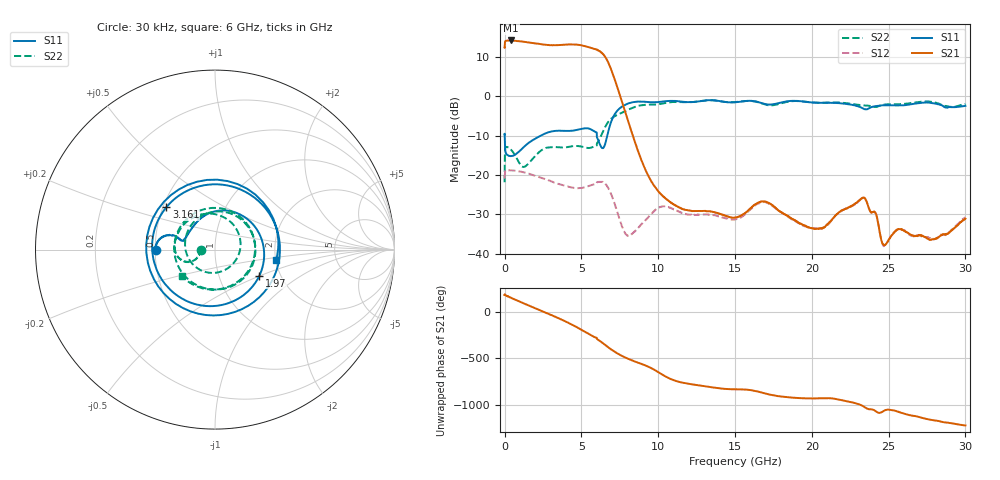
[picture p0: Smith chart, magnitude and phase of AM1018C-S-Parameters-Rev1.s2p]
# Hz S DB R 50.0
!freq dBS11 angS11 dBS21 angS21 dBS12 angS12 dBS22 angS22
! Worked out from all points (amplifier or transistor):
!   2882 points, 30 kHz to 30 GHz, reference 50 ohm
!   highest |S21| = 14.2 dB at 431.6 MHz (marker M1)
!   |S21| within 3 dB of that: start of sweep to 6.277 GHz
!   unconditionally stable (mu >= 1): start of sweep to end of sweep
!   at 1.168 MHz: K = 1.38, MAG = 12.8 dB, |S12| = -20.7 dB
!   at 1.784 GHz: K = 1.20, MAG = 14.0 dB, |S12| = -20.0 dB
!   at 30 GHz: K = 100.35, MAG = -23.2 dB, |S12| = -30.8 dB
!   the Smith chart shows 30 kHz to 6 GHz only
!   S11 on the Smith chart (normalised r, x): 30 kHz: 0.50, -0.00; 1.97 GHz: 1.56, -0.49; 3.161 GHz: 0.52, +0.28; 6 GHz: 2.00, -0.27
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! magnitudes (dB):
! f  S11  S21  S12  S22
! 30 kHz  -9.7  12.3  -20.7  -21.9
! 15.16 MHz  -11.6  13.4  -19.6  -15.0
! 40.55 MHz  -13.8  14.0  -19.0  -13.2
! 431.6 MHz  -15.2  14.2  -18.8  -13.6
! 1.191 GHz  -13.1  13.9  -19.3  -18.0
! 1.97 GHz  -10.8  13.4  -20.2  -15.3
! 3.161 GHz  -8.9  13.0  -21.8  -12.9
! 5.034 GHz  -8.3  12.9  -23.3  -12.8
! 6 GHz  -9.3  11.9  -22.2  -12.5
! 6.439 GHz  -13.1  10.6  -21.9  -8.7
! 7.189 GHz  -4.5  4.0  -27.6  -5.0
! 8.032 GHz  -1.9  -6.2  -35.5  -3.5
! 10 GHz  -1.5  -24.1  -28.3  -2.1
! 15.01 GHz  -1.5  -30.9  -31.3  -1.5
! 16.94 GHz  -2.0  -26.8  -26.9  -2.1
! 20.01 GHz  -1.6  -33.6  -33.5  -1.6
! 23.31 GHz  -3.1  -25.9  -25.9  -2.3
! 24.66 GHz  -2.3  -37.7  -38.0  -2.2
! 25.01 GHz  -2.3  -36.5  -36.5  -2.1
! 25.73 GHz  -2.3  -33.8  -33.8  -2.0
! 27.99 GHz  -1.8  -36.3  -36.4  -1.6
! 30 GHz  -2.5  -31.1  -30.8  -2.0
